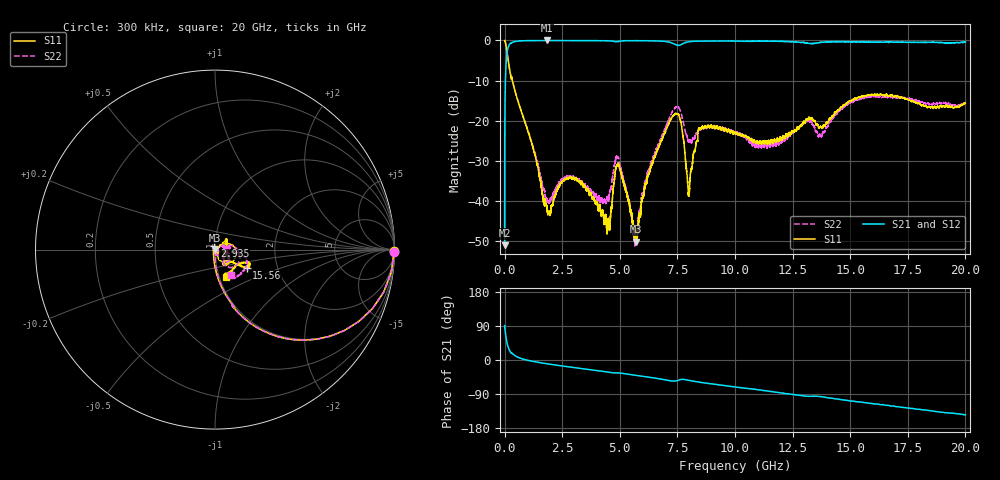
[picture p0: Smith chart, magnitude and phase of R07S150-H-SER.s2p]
!{R07S150}
!Johanson Technology Inc.
!www.johansontechnology.com
!Test Board Conditions:
!Substrate Type  RO4350B
!Substrate Thickness  10 mil
!Substrate Dk  3.66
!TL Type: GCPW
!TL Trace Width  21 mil
!TL Gap  20 mil
!Electrode orientation  Horizontal
!DUT TOPOLOGY	SERIES
!Mounting Pad LxW  16x21 mil
! Created Sat Feb  6 11:46:51 2021
# hz S ma R 50
! 2 Port Network Data from SP1.SP block
! freq  magS11  angS11  magS21  angS21  magS12  angS12  magS22  angS22
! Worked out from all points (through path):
!   20001 points, 300 kHz to 20 GHz, reference 50 ohm
!   highest |S21| = -0.01 dB at 1.833 GHz (marker M1); lowest = -51.1 dB at 300 kHz (marker M2)
!   group delay of S21, straight-line fit = 21.2 ps
!   lowest |S11| = -50.2 dB at 5.689 GHz (marker M3), VSWR 1.01, Z = 50.2 - j0.235 ohm
!   |S11| at or under -10 dB: 338.2 MHz to end of sweep
!   |S22| runs from -51.3 to 0.0 dB; largest |S21 - S12| = 0.013
!   S11 on the Smith chart (normalised r, x): 300 kHz: open; 2.935 GHz: 0.99, +0.04; 15.56 GHz: 1.39, -0.30; 20 GHz: 1.08, -0.34
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300000  0.9977 -0.5  0.002787 90.9  0.002889 90.0  1 -0.6
1.033e8  0.7149 -44.9  0.6955 45.4  0.6971 45.3  0.7151 -44.8
1.893e8  0.4853 -62.3  0.8712 28.1  0.871 28.2  0.4848 -62.3
5.583e8  0.1839 -82.2  0.9815 7.9  0.9804 7.8  0.1841 -81.4
1.8333e9  0.008339 -152.0  0.9991 -9.9  0.9974 -9.9  0.01056 -39.3
2.9353e9  0.01886 101.9  0.9953 -19.4  0.9962 -19.3  0.0198 28.3
3.3343e9  0.01655 105.0  0.9948 -22.5  0.9956 -22.5  0.01759 16.8
4.5013e9  0.005792 95.9  0.9895 -32.0  0.9894 -32.0  0.01026 -14.5
4.9073e9  0.029 -68.6  0.9668 -34.0  0.9672 -34.0  0.03489 -63.8
5.6893e9  0.003103 -49.0  0.9938 -40.6  0.9936 -40.5  0.003525 -20.3
6.1433e9  0.01621 29.7  0.9909 -44.4  0.9913 -44.4  0.01795 32.8
6.6673e9  0.04539 33.3  0.9848 -49.1  0.9855 -49.2  0.04948 25.4
7.5093e9  0.1214 -26.3  0.8712 -54.3  0.8705 -54.3  0.15 -30.3
7.9983e9  0.01173 -2.9  0.9641 -53.7  0.9628 -53.8  0.05486 -40.1
8.4873e9  0.07899 41.7  0.979 -58.8  0.9796 -58.8  0.07715 9.7
1.00003e10  0.07098 22.7  0.9821 -71.1  0.9832 -71.1  0.0685 8.6
1.15793e10  0.05718 -20.0  0.9788 -83.1  0.9793 -83.3  0.0527 20.2
1.33343e10  0.1071 -56.0  0.9136 -95.6  0.9146 -95.7  0.09401 -46.9
1.37053e10  0.08471 -55.9  0.9469 -96.5  0.9439 -96.5  0.06709 -30.2
1.55583e10  0.2035 -30.0  0.9602 -112.1  0.9598 -112.0  0.1909 -20.9
1.66673e10  0.2025 -22.6  0.9457 -119.9  0.952 -120.3  0.1993 -42.0
2e10  0.165 -67.8  0.9515 -144.8  0.9448 -144.7  0.1673 -57.6
